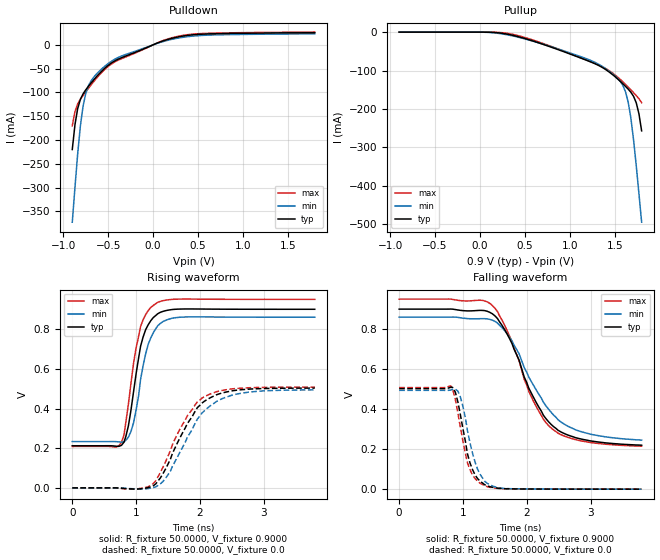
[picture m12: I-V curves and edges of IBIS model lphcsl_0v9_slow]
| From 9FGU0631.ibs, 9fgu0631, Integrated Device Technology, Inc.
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[Model]  lphcsl_0v9_slow
Model_type Output
Polarity   Non-Inverting
Enable   Active-High
Vmeas =  0.4000V
Cref =   2.0000pF
Rref =   0.0
Vref =   0.4000V
C_comp   1.1000pF   1.0000pF   1.2000pF
[Temperature Range]   25.0000   75.0000   0.0
[Voltage Range]   0.9000V   0.8600V   0.9500V
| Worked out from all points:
|   slope of the pulldown table from 0 to 0.135 V, typ, clamps not added: 14 ohm
|   slope of the pullup table from 0 to 0.135 V, typ, clamps not added: 242 ohm
|   rising waveform, R_fixture 50.0000, V_fixture 0.9000: 20-80 % time 214ps typ, 225ps min, 212ps max; typ from 0.212 V to 0.9 V
|   rising waveform, R_fixture 50.0000, V_fixture 0.0: 20-80 % time 486ps typ, 536ps min, 484ps max; typ from 0 V to 0.503 V
|   falling waveform, R_fixture 50.0000, V_fixture 0.9000: 20-80 % time 581ps typ, 653ps min, 563ps max; typ from 0.9 V to 0.22 V
|   falling waveform, R_fixture 50.0000, V_fixture 0.0: 20-80 % time 206ps typ, 218ps min, 200ps max; typ from 0.503 V to 0 V
[Pulldown]
|Voltage   I(typ)   I(min)   I(max)
-900mV    -219.9mA   -372.5mA   -170.2mA
-870mV    -167.7mA   -299.2mA   -140.4mA
-840mV    -134mA     -229.3mA   -124.2mA
-810mV    -114.7mA   -170.8mA   -114.3mA
-780mV    -103.1mA   -129mA     -106.3mA
-750mV    -94.51mA   -102.1mA   -98.78mA
-720mV    -87.03mA   -85.88mA   -91.35mA
-660mV    -73.27mA   -67.73mA   -76.97mA
-510mV    -44.58mA   -40.66mA   -46.85mA
60mV      4.726mA    3.957mA    5.199mA
330mV     18.28mA    15.74mA    19.79mA
1.8V      25.49mA    23.19mA    26.76mA
[Pullup]
|Voltage   I(typ)   I(min)   I(max)
-900mV    58.12uA    179.8uA    108.4uA
30mV      -27.1uA    -120.7uA   -3.07uA
330mV     -6.434mA   -8.091mA   -4.143mA
1.17V     -71.69mA   -67.79mA   -71.08mA
1.47V     -109.4mA   -107.2mA   -105.3mA
1.59V     -134.1mA   -138.1mA   -129.1mA
1.62V     -141mA     -154.8mA   -135.9mA
1.65V     -148.2mA   -181.8mA   -142.9mA
1.68V     -156.4mA   -223.1mA   -150.2mA
1.74V     -183.8mA   -347.1mA   -165.1mA
1.77V     -212.4mA   -420.1mA   -173.2mA
1.8V      -256.9mA   -494.7mA   -183.7mA
[Ramp]
| variable   typ   min   max
dV/dt_r  0.3016/0.5164n   0.2962/0.5704n   0.3046/0.4877n
dV/dt_f  0.4081/0.6184n   0.3688/0.6853n   0.4411/0.5951n
R_load = 50.0000
[Rising Waveform]
R_fixture= 50.0000
V_fixture= 0.9000
V_fixture_min= 0.8600
V_fixture_max= 0.9500
|time   V(typ)   V(min)   V(max)
0s        212.3mV    233.4mV    208.8mV
770ps     214.2mV    230.5mV    229.5mV
810ps     230mV      231.7mV    265.6mV
920ps     392mV      284.3mV    527.8mV
1ns       574.6mV    392.7mV    704.8mV
1.07ns    713.1mV    546.2mV    812.9mV
1.19ns    822mV      723.4mV    893.7mV
1.34ns    877.7mV    817.3mV    935mV
1.73ns    901.3mV    860.5mV    951.4mV
3.8ns     899.9mV    860mV      949.9mV
[Rising Waveform]
R_fixture= 50.0000
V_fixture= 0.0
V_fixture_min= 0.0
V_fixture_max= 0.0
|time   V(typ)   V(min)   V(max)
0s        0V         0V         0V
960ps     -5.661mV   -4.414mV   -6.434mV
1.23ns    5.448mV    -1.222mV   11.86mV
1.31ns    20.53mV    5.226mV    36.4mV
1.46ns    94.27mV    47.43mV    130.5mV
1.8ns     321.9mV    252.5mV    361.3mV
1.96ns    404.4mV    346.6mV    433.1mV
2.15ns    451.9mV    410.3mV    471.7mV
2.65ns    494.6mV    476.9mV    502.6mV
3.8ns     502.7mV    493.7mV    507.6mV
[Falling Waveform]
R_fixture= 50.0000
V_fixture= 0.9000
V_fixture_min= 0.8600
V_fixture_max= 0.9500
|time   V(typ)   V(min)   V(max)
0s        900mV      860mV      950mV
1.42ns    884.1mV    848.8mV    929.1mV
1.54ns    853.4mV    830.7mV    888.6mV
1.73ns    752.8mV    760.1mV    764.6mV
1.88ns    644.8mV    676.4mV    642.1mV
2.03ns    506.2mV    561.4mV    490.6mV
2.34ns    337.7mV    400.4mV    318.3mV
2.53ns    287mV      337.2mV    273.6mV
2.8ns     254.5mV    292.8mV    244.9mV
3.8ns     219.9mV    245.3mV    214.9mV
[Falling Waveform]
R_fixture= 50.0000
V_fixture= 0.0
V_fixture_min= 0.0
V_fixture_max= 0.0
|time   V(typ)   V(min)   V(max)
0s        502.9mV    494.1mV    507.7mV
810ps     509.4mV    495.6mV    516.5mV
880ps     485.3mV    500.1mV    449.8mV
920ps     436.7mV    490.6mV    382.3mV
1ns       301.4mV    412.3mV    239.2mV
1.11ns    131.5mV    232.3mV    97.74mV
1.23ns    52.56mV    98.73mV    39.7mV
1.34ns    22.24mV    39.69mV    17mV
1.69ns    2.043mV    3.046mV    1.708mV
3.8ns     65.31uV    100.4uV    50.85uV
